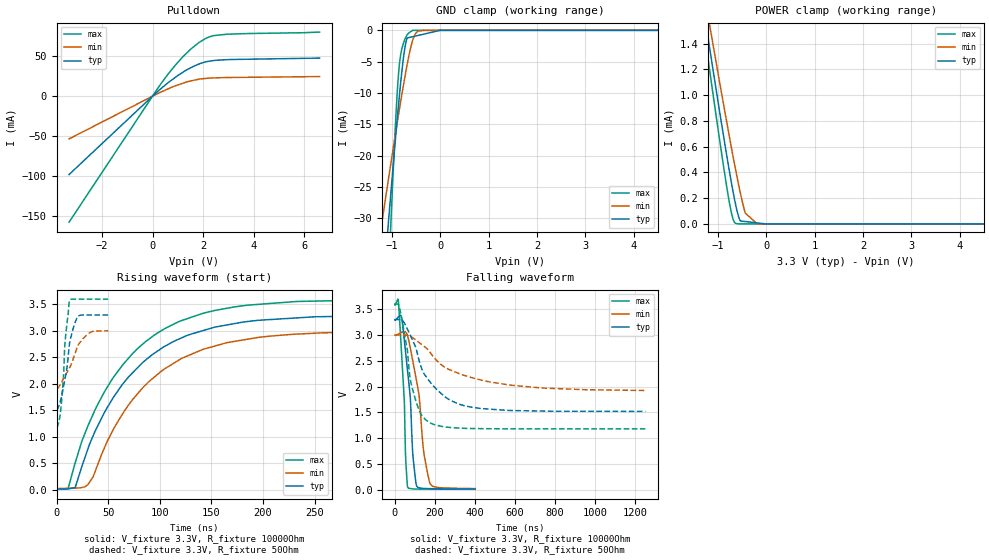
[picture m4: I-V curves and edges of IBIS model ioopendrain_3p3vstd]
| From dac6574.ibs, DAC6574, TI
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|   ioopendrain_3p3vstd Model
[Model]   ioopendrain_3p3vstd
Model_type   I/O_open_drain
Polarity   Non-Inverting
Enable   Active-Low
Vinl = 0.99
Vinh = 2.31
Vmeas = 1.65
Vref = 3.3
Cref = 400pF
Rref = 10000
|   typ   min   max
|   (nom PVT)   (Fast PVT)   (slow PVT)
|Average
C_comp   5.118e-12   5.087e-12   5.165e-12
|ON state : BUFFER OUTPUT TURNED LOW
|C_comp   5.602e-10   5.027e-10   5.985e-10
|OFF state: BUFFER in HIGH IMPEDANCE
|C_comp   5.118e-12   5.087e-12   5.165e-12
| Where nom  PVT is Nominal Process, 3.3V, 25C
|   Fast PVT is Strong Process,  3.6V, -40C
|   Slow PVT is Weak Process,   3V, 105C
[Model spec]
|   typ   min   max
Vinl   0.99   0.9   1.08
Vinh   2.31   2.1   2.52
[Voltage Range]   3.3   3   3.6
|Ambient Temperature   25   105   -40
|Junction Temperature
[Temperature Range]   25   105   -40
[Pullup Reference]   3.3   3   3.6
[Pulldown Reference]   0   0   0
[Power Clamp Reference]   3.3   3   3.6
[GND Clamp Reference]   0   0   0
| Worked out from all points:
|   slope of the pulldown table from 0 to 0.495 V, typ, clamps not added: 36.2 ohm
|   GND clamp passes 1 mA (typ) near -0.56 V on its own axis
|   POWER clamp passes 1 mA (typ) near -1.02 V on its own axis
|   falling waveform, V_fixture 3.3V, R_fixture 10000Ohm: 20-80 % time 35.8ns typ, 54.7ns min, 22.9ns max; typ from 3.3 V to 0.011 V
|   rising waveform, V_fixture 3.3V, R_fixture 10000Ohm: 20-80 % time 71ns typ, 72.2ns min, 70.6ns max; typ from 0.011 V to 3.3 V
|   falling waveform, V_fixture 3.3V, R_fixture 50Ohm: 20-80 % time 145ns typ, 273ns min, 66.4ns max; typ from 3.3 V to 1.52 V
|   rising waveform, V_fixture 3.3V, R_fixture 50Ohm: 20-80 % time 8.67ns typ, 15ns min, 5.15ns max; typ from 1.52 V to 3.3 V
[Pulldown]
|   Voltage   I(typ)   I(min)   I(max)
-3.3V     -97.88mA   -53.33mA   -157.4mA
318mV     9.006mA    5.005mA    14.9mA
876mV     22.96mA    12.66mA    37.86mA
1.204V    29.99mA    16.21mA    49.42mA
1.52V     35.68mA    19.08mA    59.08mA
1.823V    40.01mA    21.17mA    66.75mA
2.262V    43.76mA    22.62mA    74.29mA
2.942V    45.57mA    23.31mA    77.37mA
6.6V      47.55mA    24.48mA    80.03mA
[GND Clamp]
|   Voltage   I(typ)   I(min)   I(max)
-3.3V     -246.7mA   -140.1mA   -463.1mA
-1.269V   -49.35mA   -33.72mA   -76.76mA
-1.208V   -43.43mA   -30.6mA    -65.2mA
-1.072V   -30.43mA   -23.65mA   -39.58mA
-1.047V   -28.13mA   -22.41mA   -35.08mA
-1.021V   -25.74mA   -21.13mA   -30.4mA
-913.2mV  -15.96mA   -15.79mA   -12.69mA
-837.6mV  -9.656mA   -12.16mA   -4.795mA
-706.2mV  -1.692mA   -6.233mA   -973.9uA
-574.8mV  -1.018mA   -1.632mA   0A
-330mV    -584.6uA   0A         0A
6.6V      0A         0A         0A
[POWER Clamp]
|   Voltage   I(typ)   I(min)   I(max)
-3.3V     6.651mA    6.278mA    7.033mA
-1.313V   1.712mA    1.855mA    1.577mA
-1.247V   1.552mA    1.712mA    1.401mA
-1.154V   1.327mA    1.51mA     1.152mA
-873.6mV  662.5uA    910uA      425.5uA
-762mV    411.2uA    678.4uA    166.8uA
-690mV    259.4uA    532.3uA    42.61uA
-621.6mV  131.7uA    399.4uA    2.885uA
-534.6mV  22.99uA    239.9uA    49.42nA
-432mV    18.58uA    83.42uA    39.92nA
-183mV    7.869uA    124nA      16.87nA
6.6V      0A         0A         0A
[Ramp]
R_load = 10000
|   typ   min   max
dV/dt_r   1.97329/7.09099e-08   1.78903/7.15706e-08   2.15552/7.05508e-08
dV/dt_f   1.9733/3.5723e-08   1.78902/5.4664e-08   2.15552/2.28389e-08
[Falling Waveform]
V_fixture = 3.3V
V_fixture_min = 3V
V_fixture_max = 3.6V
R_fixture = 10000Ohm
|   Time   V(typ)   V(min)   V(max)
0s        3.3V       3V         3.6V
18.91ns   3.359V     3.022V     3.594V
46.91ns   2.905V     3.066V     1.731V
53.06ns   2.679V     3.06V      679.3mV
63.62ns   2.29V      2.975V     50.39mV
88.78ns   720.8mV    2.507V     12.19mV
108.5ns   70.72mV    2.101V     10.18mV
142.2ns   20.54mV    785.2mV    8.787mV
177ns     17.38mV    105.1mV    8.325mV
400ns     11.17mV    18.3mV     7.473mV
[Rising Waveform]
V_fixture = 3.3V
V_fixture_min = 3V
V_fixture_max = 3.6V
R_fixture = 10000Ohm
|   Time   V(typ)   V(min)   V(max)
0s        11.17mV    18.28mV    7.473mV
11.28ns   12.63mV    24.88mV    23.46mV
18.08ns   37.88mV    28.86mV    506.5mV
35.33ns   1.011V     237mV      1.42V
54.65ns   1.729V     1.122V     2.11V
84.17ns   2.414V     1.939V     2.762V
120ns     2.857V     2.465V     3.186V
165.3ns   3.112V     2.778V     3.427V
229.8ns   3.241V     2.936V     3.551V
500ns     3.3V       3V         3.6V
[Falling Waveform]
V_fixture = 3.3V
V_fixture_min = 3V
V_fixture_max = 3.6V
R_fixture = 50Ohm
|   Time   V(typ)   V(min)   V(max)
0s        3.3V       3V         3.6V
25.08ns   3.299V     3V         3.498V
62.23ns   3.116V     2.994V     2.709V
77.05ns   2.994V     2.976V     2.129V
101.7ns   2.785V     2.912V     1.758V
137.1ns   2.313V     2.806V     1.425V
175.3ns   2.09V      2.665V     1.296V
274.4ns   1.738V     2.324V     1.206V
424.7ns   1.575V     2.131V     1.183V
1.25us    1.517V     1.923V     1.178V
[Rising Waveform]
V_fixture = 3.3V
V_fixture_min = 3V
V_fixture_max = 3.6V
R_fixture = 50Ohm
|   Time   V(typ)   V(min)   V(max)
0s        1.517V     1.917V     1.178V
2.198ns   1.577V     1.94V      1.275V
4.203ns   1.705V     2.006V     1.526V
6.676ns   1.936V     2.092V     2.115V
8.195ns   2.092V     2.146V     2.771V
10.05ns   2.292V     2.213V     3.13V
12.56ns   2.756V     2.302V     3.559V
20.54ns   3.273V     2.716V     3.599V
33.35ns   3.299V     2.978V     3.599V
50ns      3.3V       3V         3.6V
